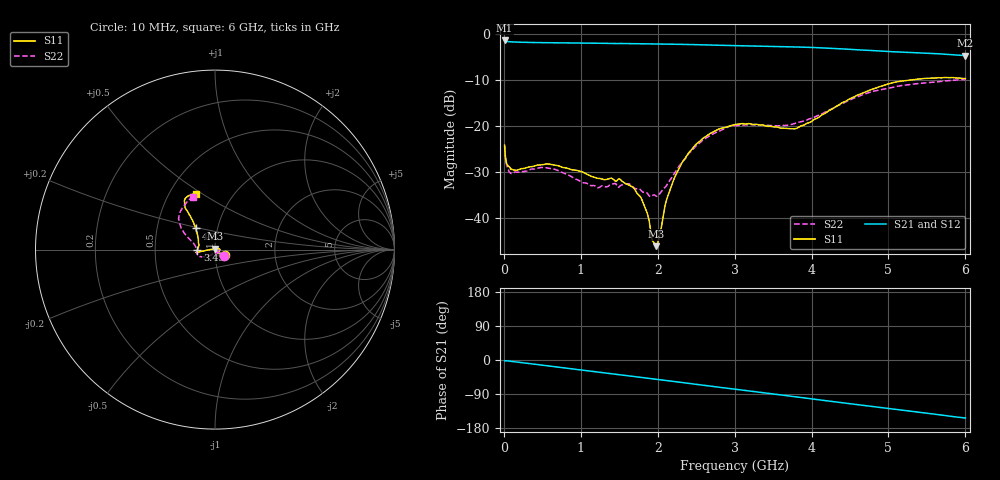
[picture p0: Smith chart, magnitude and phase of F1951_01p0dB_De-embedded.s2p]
! Integrated Device Technology
! Corporate Headquarters
! 6024 Silver Creek Valley Road
! San Jose, CA 95138  USA
! Phone:  1-408-284-8200
! Toll Free:  1-800-223-1366
! Webpage:  http://www.idt.com/
! Timing and RF Division
! 515 Groton Road, Suite 102
! Westford, MA 01886-6024
! Device:  F1951
! Description: 6-bit 0.5 dB Digital Step Attenuator
! Frequency:  100.0 -  4000.00 MHz
! Package:  4x4 mm Thin QFN Plastic Package: 24 pin
! Ports:  2 RF, 6 DC
!  Pin  1  = NC
!  Pin  2  = RF1  =  Port 1
!  Pin  3  = GND
!  Pin  4  = NC
!  Pin  5  = Serial Data Out (SDO)
!  Pin  6  = NC
!  Pin  7  = Reset Bar ( RSTb)
!  Pin  8  = Clock (CLK)
!  Pin  9  = Chip Select Bar (CSb)
!  Pin 10  = NC
!  Pin 11  = Serial Data In (SDI)
!  Pin 12  = NC
!  Pin 13  = NC
!  Pin 14  = VDD
!  Pin 15  = NC
!  Pin 16  = GND
!  Pin 17  = RF2  =  Port 2
!  Pin 18  = NC
!  Pin 19  = GND
!  Pin 20  = GND
!  Pin 21  = GND
!  Pin 22  = GND
!  Pin 23  = GND
!  Pin 24  = GND
! State:  2
! Atten State:  1.0 dB
! Voltage:  +3.30 Volts
! Current:  0.472 mA
! Data:  The device was measured on a F195X evaluation board which has
!  individual transmission lines to the RF pins.  Data was collected
!  de-embedded using a Automatic Fixture Removal [AFR] (Keysight Technologies).
!  The reference plane is the edge of the package pin.
! Misc:  Lot Code  1225BCA
!  Action Tracker AT0399
! Date Measured:  2018-09-13
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# GHz S dB R 50
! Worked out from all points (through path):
!   600 points, 10 MHz to 6 GHz, reference 50 ohm
!   highest |S21| = -1.42 dB at 10 MHz (marker M1); lowest = -4.7 dB at 6 GHz (marker M2)
!   group delay of S21, straight-line fit = 70.7 ps
!   lowest |S11| = -46.2 dB at 1.98 GHz (marker M3), VSWR 1.01, Z = 49.9 + j0.481 ohm
!   |S11| at or under -10 dB: start of sweep to 5.302 GHz
!   |S22| runs from -35.4 to -9.9 dB; largest |S21 - S12| = 0.00095
!   S11 on the Smith chart (normalised r, x): 10 MHz: 1.11, -0.07; 3.45 GHz: 0.82, -0.01; 4.3 GHz: 0.79, +0.19; 6 GHz: 0.68, +0.47
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0.01  -24.21 -30.3  -1.42 -2.3  -1.42 -2.3  -24.35 -33.4
0.05  -28.62 -31.9  -1.67 -2.4  -1.67 -2.4  -29.34 -34.3
0.1  -29.47 -39.2  -1.72 -3.6  -1.73 -3.6  -30.40 -41.8
0.55  -28.32 -67.9  -1.90 -14.8  -1.90 -14.8  -29.13 -75.1
1.01  -29.97 -43.9  -2.00 -26.3  -2.00 -26.3  -32.26 -52.9
1.51  -31.64 4.0  -2.08 -38.6  -2.08 -38.6  -33.12 -5.8
1.68  -33.44 13.7  -2.10 -43.0  -2.11 -43.0  -33.32 -9.2
1.81  -36.76 24.1  -2.13 -46.4  -2.13 -46.4  -34.48 -23.1
1.87  -39.39 26.5  -2.15 -47.9  -2.15 -47.9  -34.82 -33.5
1.94  -45.24 61.4  -2.16 -49.7  -2.16 -49.7  -35.08 -53.5
1.98  -46.22 99.8  -2.17 -50.7  -2.17 -50.7  -35.32 -62.1
2.01  -44.90 136.9  -2.18 -51.5  -2.18 -51.5  -35.21 -72.3
2.13  -35.38 173.7  -2.21 -54.6  -2.21 -54.6  -32.63 -102.2
2.34  -27.46 -175.3  -2.28 -60.1  -2.28 -60.1  -27.54 -130.9
2.61  -22.50 -172.6  -2.38 -67.1  -2.38 -67.1  -22.87 -146.3
3.01  -19.69 -170.2  -2.54 -77.2  -2.54 -77.1  -19.95 -160.9
3.45  -20.10 -177.5  -2.68 -88.3  -2.69 -88.3  -19.92 -174.0
3.78  -20.66 163.8  -2.83 -96.9  -2.84 -96.8  -19.49 174.0
4.01  -18.92 146.0  -2.94 -102.9  -2.94 -102.8  -18.32 165.2
4.3  -15.98 132.2  -3.16 -110.4  -3.16 -110.3  -15.98 156.8
5.01  -10.84 125.4  -3.84 -128.1  -3.84 -128.1  -11.82 141.2
6  -9.71 109.3  -4.70 -153.1  -4.70 -153.1  -9.91 112.4
